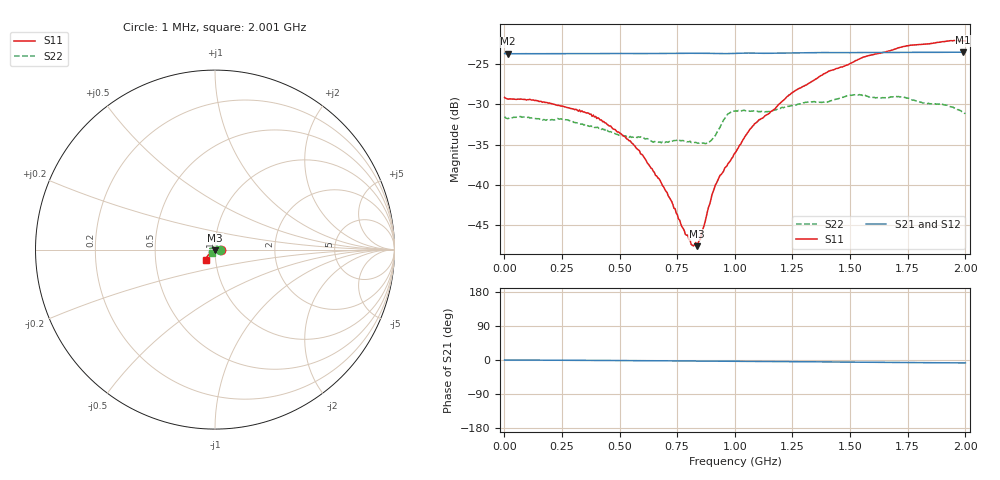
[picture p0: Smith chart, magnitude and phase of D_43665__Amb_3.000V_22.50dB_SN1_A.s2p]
! device id: 43665_
! dir: \\malibu\benchdata\1_engineers\tn_data\43665_75ohm\new\sparar\43665_\amb\3p000v\22p50db
! Serial: 1
! Insertion: A
! Temp: Amb
! VDD: 3.000V
! Attenuation Step: 22.50dB
! IDD: 1.452686e+00mA
! FILE NAME
! DATE 03-27-2009 08:38:53
! CORRECTED  DATA
#  Hz  S  RI  R  75
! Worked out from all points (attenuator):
!   401 points, 1 MHz to 2.001 GHz, reference 75 ohm
!   highest |S21| = -23.54 dB at 1.991 GHz (marker M1); lowest = -23.7 dB at 16 MHz (marker M2)
!   lowest |S11| = -47.6 dB at 836 MHz (marker M3), VSWR 1.01, Z = 75.1 - j0.622 ohm
!   |S11| at or under -10 dB: start of sweep to end of sweep
!   |S22| runs from -34.9 to -28.8 dB; largest |S21 - S12| = 0.00031
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1000000  0.0348 -0.000318  0.0653 -5.63e-05  0.0651 -0.000143  0.0265 -0.000222
1.6e7  0.034 6.27e-05  0.065 -5.66e-05  0.0651 -8.43e-05  0.0257 0.000745
2.41e8  0.0309 0.00169  0.0651 -0.000727  0.0652 -0.000702  0.0223 0.0125
3.36e8  0.0288 0.00189  0.0651 -0.00105  0.0652 -0.00103  0.0173 0.0164
4.16e8  0.0251 0.00251  0.0652 -0.00127  0.0652 -0.00121  0.0133 0.0181
5.46e8  0.0187 0.00128  0.0652 -0.00189  0.0653 -0.00181  0.00522 0.0193
6.71e8  0.0109 -0.000777  0.0653 -0.00223  0.0653 -0.00215  -0.0027 0.0182
8.11e8  0.00214 -0.00371  0.0654 -0.00301  0.0654 -0.00288  -0.0118 0.014
8.36e8  0.000513 -0.00414  0.0654 -0.00313  0.0655 -0.003  -0.0133 0.0124
8.56e8  -0.0013 -0.00484  0.0654 -0.00326  0.0654 -0.00312  -0.0145 0.011
8.86e8  -0.00374 -0.00623  0.0653 -0.00342  0.0654 -0.00332  -0.0163 0.00883
9.21e8  -0.00629 -0.00812  0.0652 -0.00363  0.0652 -0.00345  -0.02 0.00639
9.61e8  -0.00885 -0.00942  0.0651 -0.00357  0.0652 -0.00341  -0.0256 0.00643
1.001e9  -0.012 -0.0102  0.0653 -0.00357  0.0653 -0.00339  -0.0276 0.00799
1.096e9  -0.0196 -0.0146  0.0654 -0.00432  0.0655 -0.00414  -0.0284 0.00396
1.246e9  -0.0295 -0.0224  0.0656 -0.0048  0.0657 -0.00461  -0.0307 -0.00444
1.336e9  -0.0343 -0.0273  0.0658 -0.00532  0.066 -0.00511  -0.0315 -0.00874
1.521e9  -0.044 -0.0387  0.0658 -0.00649  0.066 -0.0064  -0.032 -0.0171
1.671e9  -0.0484 -0.0475  0.0659 -0.00734  0.066 -0.00724  -0.0288 -0.0196
1.901e9  -0.051 -0.058  0.0659 -0.00849  0.066 -0.00831  -0.0234 -0.0212
1.991e9  -0.0497 -0.0604  0.0659 -0.00888  0.0661 -0.00893  -0.0197 -0.0203
2.001e9  -0.0495 -0.0602  0.0659 -0.00891  0.066 -0.00896  -0.0194 -0.0197
